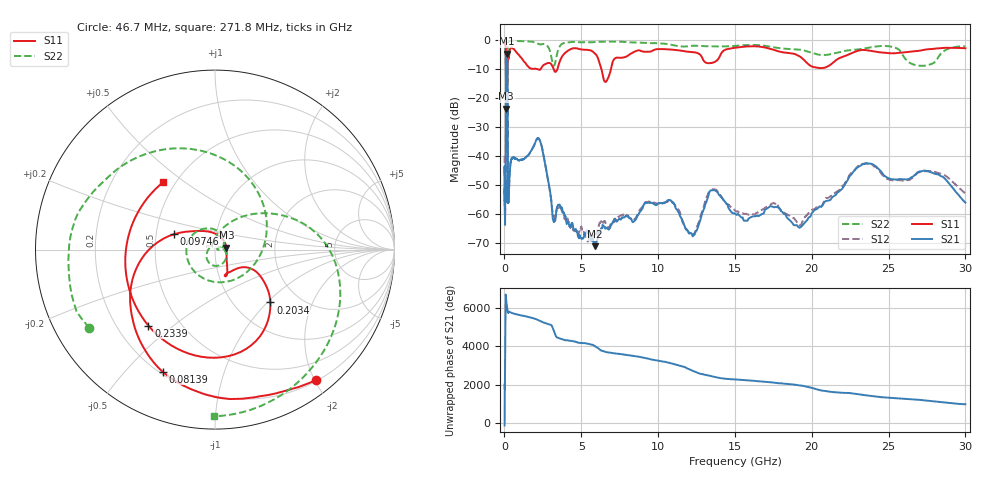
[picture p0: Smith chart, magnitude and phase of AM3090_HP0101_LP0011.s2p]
! Date/Time: Thu, Feb 28, 2019 1:58 PM
! Network Analyzer: Agilent Technologies E8364B Rev: A.07.50.67
! Sweep from 0.010 to 30.000 GHz, 1601 Points, Sweep Type: LOG
! Power Supply: 5.023 V, 0.002 A
# Hz S DB R 50
!freq MagS11 AngS11 MagS21 AngS21 MagS12 AngS12 MagS22 AngS22
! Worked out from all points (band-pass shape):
!   1601 points, 10 MHz to 30 GHz, reference 50 ohm
!   highest |S21| = -4.76 dB at 145.4 MHz (marker M1); lowest = -71.2 dB at 5.87 GHz (marker M2)
!   |S21| within 3 dB of the highest: 106.5 MHz to 188.7 MHz (82.16 MHz wide, 55.7 % of centre)
!   lowest |S11| = -23.8 dB at 105.1 MHz (marker M3), VSWR 1.14, Z = 56.8 + j1.31 ohm
!   |S11| at or under -10 dB: 2.138 GHz to 2.359 GHz (220.6 MHz wide, 9.81 % of centre); 3.197 GHz to 3.449 GHz (251.4 MHz wide, 7.57 % of centre); 6.308 GHz to 6.932 GHz (624.5 MHz wide, 9.43 % of centre)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
!   |S22| runs from -38.4 to -0.2 dB; largest |S21 - S12| = 0.013
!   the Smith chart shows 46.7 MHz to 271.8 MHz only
!   S11 on the Smith chart (normalised r, x): 46.7 MHz: 0.22, -2.02; 81.39 MHz: 0.21, -0.64; 97.46 MHz: 0.62, +0.11; 203.4 MHz: 1.45, -1.04; 233.9 MHz: 0.33, -0.41; 271.8 MHz: 0.43, +0.41
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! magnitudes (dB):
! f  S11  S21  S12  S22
! 10 MHz  -0.2  -46.7  -40.0  -0.6
! 38.04 MHz  -0.5  -59.6  -60.9  -1.4
! 46.7 MHz  -0.8  -50.4  -49.2  -1.7
! 81.39 MHz  -2.6  -46.7  -47.7  -5.4
! 97.46 MHz  -12.3  -15.2  -15.2  -15.2
! 105.1 MHz  -23.8  -8.3  -8.4  -16.7
! 131.6 MHz  -16.2  -5.0  -4.9  -38.4
! 144.7 MHz  -16.6  -4.8  -4.7  -24.9
! 145.4 MHz  -16.6  -4.8  -4.7  -24.4
! 180.3 MHz  -14.5  -6.3  -6.3  -30.3
! 203.4 MHz  -7.4  -16.7  -16.7  -10.0
! 233.9 MHz  -5.0  -55.0  -54.8  -1.5
! 271.8 MHz  -6.5  -53.6  -55.3  -0.6
! 550.5 MHz  -2.9  -40.7  -40.7  -0.3
! 2.084 GHz  -10.0  -34.4  -34.4  -1.0
! 3.204 GHz  -10.1  -62.8  -60.7  -8.9
! 5.87 GHz  -4.6  -71.2  -66.8  -0.7
! 7.926 GHz  -5.7  -60.8  -60.5  -0.7
! 13.74 GHz  -7.4  -52.1  -51.7  -2.2
! 19.12 GHz  -5.4  -64.6  -63.7  -3.3
! 23.59 GHz  -3.5  -42.6  -42.7  -2.8
! 30 GHz  -2.8  -56.1  -53.1  -2.2
